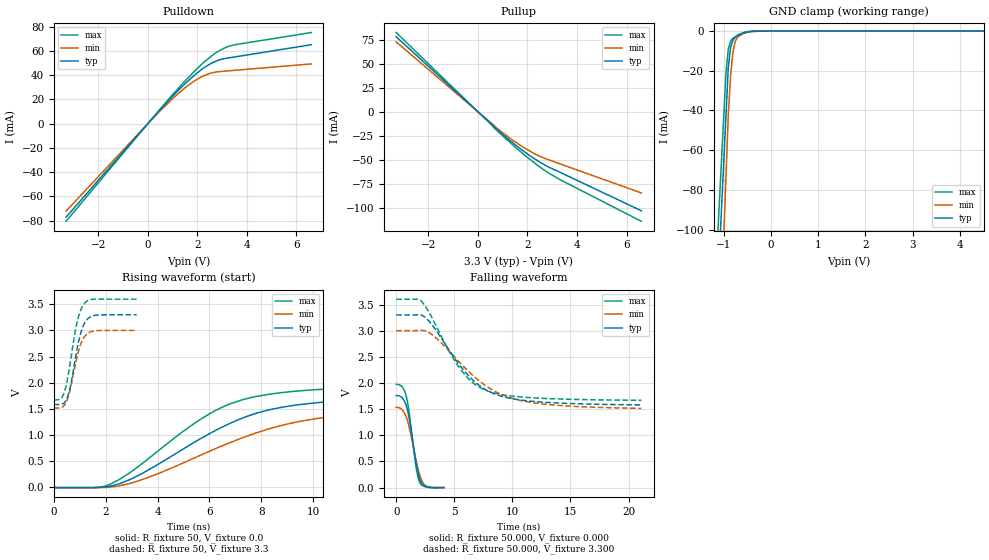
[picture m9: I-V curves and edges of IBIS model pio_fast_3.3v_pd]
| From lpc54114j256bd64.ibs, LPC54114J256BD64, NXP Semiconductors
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[Model]   pio_fast_3.3v_pd
Model_type I/O
Vinl=8.000E-01
Vinh=2.000E+00
Vref=0.000E+00
Rref=1.000E+06
Cref=2.000E-11
Vmeas=1.650E+00
C_comp   9.060E-12   8.700E-12   9.420E-12
[Voltage Range]   3.300E+00   3.000E+00   3.600E+00
[POWER Clamp Reference]   3.300E+00   3.000E+00   3.600E+00
[GND Clamp Reference]   0.000E+00   0.000E+00   0.000E+00
[Pullup Reference]   3.300E+00   3.000E+00   3.600E+00
[Pulldown Reference]   0.000E+00   0.000E+00   0.000E+00
[Temperature Range]   25   105   -40
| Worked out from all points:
|   slope of the pulldown table from 0 to 0.495 V, typ, clamps not added: 43.7 ohm
|   slope of the pullup table from 0 to 0.495 V, typ, clamps not added: 42.9 ohm
|   GND clamp passes 1 mA (typ) near -0.58 V on its own axis
|   rising waveform, R_fixture 50, V_fixture 0.0: 20-80 % time 4.01ns typ, 4.87ns min, 3.42ns max; typ from -0.007 V to 1.75 V
|   falling waveform, R_fixture 50.000, V_fixture 0.000: 20-80 % time 778ps typ, 900ps min, 693ps max; typ from 1.76 V to 0.001 V
|   rising waveform, R_fixture 50, V_fixture 3.3: 20-80 % time 406ps typ, 410ps min, 403ps max; typ from 1.58 V to 3.3 V
|   falling waveform, R_fixture 50.000, V_fixture 3.300: 20-80 % time 3.75ns typ, 4.6ns min, 3.19ns max; typ from 3.3 V to 1.58 V
[GND Clamp]
-3.3V     -1.216A    -1.571A    -1.123A
-950mV    -43.37mA   -74.42mA   -21.6mA
-900mV    -18.43mA   -42.58mA   -9.201mA
-850mV    -8.133mA   -22.12mA   -4.954mA
-800mV    -4.528mA   -10.24mA   -3.565mA
-750mV    -3.154mA   -4.987mA   -2.774mA
-700mV    -2.303mA   -3.029mA   -1.982mA
-600mV    -1.145mA   -1.463mA   -880.3uA
-400mV    -198.5uA   -152.7uA   -64.24uA
-200mV    -33.8uA    -31.76uA   -14.46uA
6.6V      135.5uA    140.2uA    126.4uA
[Power Clamp]
-3.3V     0A         0A         0A
0V        0A         0A         0A
3.3V      0A         0A         0A
6.6V      0A         0A         0A
[Pullup]
-3.3V     78.3mA     72.94mA    82.7mA
720mV     -17.43mA   -16.13mA   -18.38mA
1.36V     -31.35mA   -28.83mA   -33.53mA
1.82V     -40.62mA   -36.76mA   -43.91mA
2.5V      -52.53mA   -46.42mA   -57.65mA
3.22V     -62.03mA   -53.52mA   -69.47mA
6.6V      -103.4mA   -84.74mA   -114.4mA
[Pulldown]
-3.3V     -77.06mA   -72.09mA   -80.46mA
140mV     3.263mA    3.027mA    3.421mA
1.04V     23.4mA     21.38mA    24.81mA
1.46V     32mA       28.83mA    34.24mA
1.9V      40.22mA    35.44mA    43.55mA
2.22V     45.34mA    39.08mA    49.76mA
2.64V     50.5mA     42.1mA     56.82mA
3.12V     53.7mA     43.29mA    62.54mA
3.54V     55.09mA    44.01mA    65.14mA
6.6V      65.07mA    49.25mA    75.08mA
[Rising Waveform]
R_fixture = 50
V_fixture = 0.0
V_fixture_min = 0.0
V_fixture_max = 0.0
0s        -6.972mV   -11.77mV   -15.61mV
1.65ns    -6.031mV   -11.97mV   -9.955mV
2.2ns     18.82mV    -80.67uV   60.55mV
3.35ns    244.8mV    133.1mV    428.3mV
5.9ns     994.4mV    663.1mV    1.373V
6.8ns     1.222V     850.9mV    1.595V
7.8ns     1.413V     1.036V     1.735V
9.5ns     1.581V     1.26V      1.844V
11.85ns   1.674V     1.403V     1.905V
20.45ns   1.751V     1.522V     1.955V
[Falling Waveform]
R_fixture = 50.000
V_fixture = 0.000
V_fixture_min = 0.000
V_fixture_max = 0.000
|  time   V(typ)   V(min)   V(max)
0s        1.759V     1.535V     1.974V
550ps     1.707V     1.476V     1.916V
900ps     1.539V     1.329V     1.713V
1.15ns    1.28V      1.127V     1.376V
1.7ns     496.4mV    532.2mV    405.4mV
1.85ns    319.2mV    383.8mV    223.9mV
2ns       186.6mV    258.9mV    113.1mV
2.25ns    67.95mV    113.6mV    40.38mV
2.55ns    23.67mV    35.12mV    14.3mV
4.1ns     665uV      641.2uV    232uV
[Rising Waveform]
R_fixture = 50
V_fixture = 3.3
V_fixture_min = 3.0
V_fixture_max = 3.6
0s        1.581V     1.514V     1.67V
300ps     1.587V     1.525V     1.711V
400ps     1.612V     1.559V     1.806V
500ps     1.688V     1.647V     1.996V
650ps     1.957V     1.914V     2.438V
900ps     2.65V      2.506V     3.163V
1.05ns    2.971V     2.756V     3.408V
1.2ns     3.154V     2.893V     3.529V
1.6ns     3.291V     2.993V     3.6V
3.2ns     3.3V       3V         3.6V
[Falling Waveform]
R_fixture = 50.000
V_fixture = 3.300
V_fixture_min = 3.000
V_fixture_max = 3.600
|  time   V(typ)   V(min)   V(max)
0s        3.3V       3V         3.6V
2.2ns     3.295V     3.007V     3.555V
3.2ns     3.078V     2.905V     3.196V
4.5ns     2.646V     2.624V     2.624V
5.4ns     2.36V      2.408V     2.303V
6.5ns     2.079V     2.164V     2.023V
7.65ns    1.878V     1.957V     1.866V
9.3ns     1.733V     1.758V     1.771V
11.7ns    1.651V     1.627V     1.718V
21.1ns    1.581V     1.514V     1.67V
[Ramp]
dV/dt_r   1.0546E+00/4.0018E-09   9.2039E-01/4.8626E-09   1.1824E+00/3.4156E-09
dV/dt_f   1.0315E+00/3.7458E-09   8.9139E-01/4.5835E-09   1.1580E+00/3.1818E-09
R_load = 50
